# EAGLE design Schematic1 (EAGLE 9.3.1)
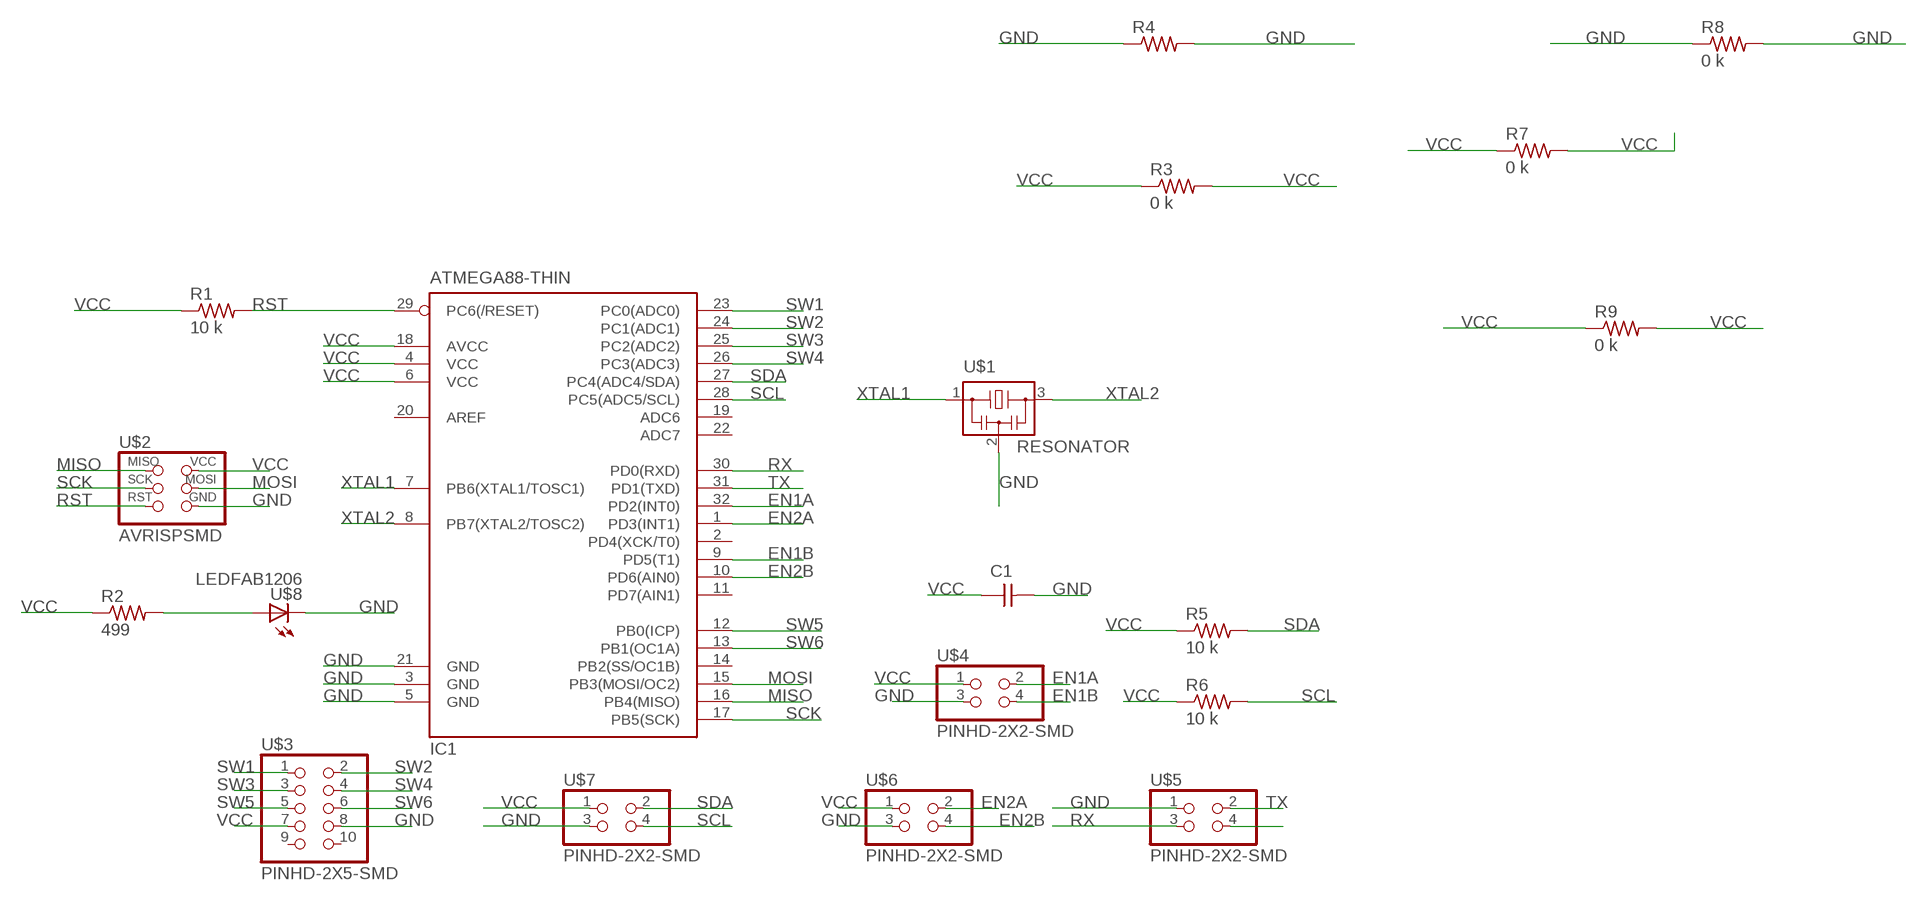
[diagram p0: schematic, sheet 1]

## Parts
C1  CAP-UNPOLARIZEDFAB  [C1206FAB]
IC1  ATMEGA88-THIN  [TQFP32-08THIN]
R1  10 k  RES-US1206FAB  [R1206FAB]
R2  499  RES-US1206FAB  [R1206FAB]
R3  0 k  RES-US1206FAB  [R1206FAB]
R4  RES-US1206FAB  [R1206FAB]
R5  10 k  RES-US1206FAB  [R1206FAB]
R6  10 k  RES-US1206FAB  [R1206FAB]
R7  0 k  RES-US1206FAB  [R1206FAB]
R8  0 k  RES-US1206FAB  [R1206FAB]
R9  0 k  RES-US1206FAB  [R1206FAB]
U$1  RESONATOR  [EFOBM]
U$2  AVRISPSMD  [2X03SMD]
U$3  PINHD-2X5-SMD  [2X05SMD]
U$4  PINHD-2X2-SMD  [2X02SMD]
U$5  PINHD-2X2-SMD  [2X02SMD]
U$6  PINHD-2X2-SMD  [2X02SMD]
U$7  PINHD-2X2-SMD  [2X02SMD]
U$8  LEDFAB1206  [LED1206FAB]

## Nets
EN1A: IC1.32(PD2(INT0)) U$4.2
EN1B: IC1.9(PD5(T1)) U$4.4
EN2A: IC1.1(PD3(INT1)) U$6.2
EN2B: IC1.10(PD6(AIN0)) U$6.4
GND: C1.2 IC1.3(GND) IC1.5(GND) IC1.21(GND) R4.1 R4.2 R8.1 R8.2 U$1.2 U$2.6(GND) U$3.8 U$4.3 U$5.1 U$6.3 U$7.3 U$8.2(C)
MISO: IC1.16(PB4(MISO)) U$2.1(MISO)
MOSI: IC1.15(PB3(MOSI/OC2)) U$2.4(MOSI)
N$1: R2.2 U$8.1(A)
N$16: U$5.4
RST: IC1.29(PC6(/RESET)) R1.2 U$2.5(RST)
RX: IC1.30(PD0(RXD)) U$5.3
SCK: IC1.17(PB5(SCK)) U$2.3(SCK)
SCL: IC1.28(PC5(ADC5/SCL)) R6.2 U$7.4
SDA: IC1.27(PC4(ADC4/SDA)) R5.2 U$7.2
SW1: IC1.23(PC0(ADC0)) U$3.1
SW2: IC1.24(PC1(ADC1)) U$3.2
SW3: IC1.25(PC2(ADC2)) U$3.3
SW4: IC1.26(PC3(ADC3)) U$3.4
SW5: IC1.12(PB0(ICP)) U$3.5
SW6: IC1.13(PB1(OC1A)) U$3.6
TX: IC1.31(PD1(TXD)) U$5.2
VCC: C1.1 IC1.4(VCC) IC1.6(VCC) IC1.18(AVCC) R1.1 R2.1 R3.1 R3.2 R5.1 R6.1 R7.1 R7.2 R9.1 R9.2 U$2.2(VCC) U$3.7 U$4.1 U$6.1 U$7.1
XTAL1: IC1.7(PB6(XTAL1/TOSC1)) U$1.1
XTAL2: IC1.8(PB7(XTAL2/TOSC2)) U$1.3
Unconnected: IC1.2(PD4(XCK/T0)) IC1.11(PD7(AIN1)) IC1.14(PB2(SS/OC1B)) IC1.19(ADC6) IC1.20(AREF) IC1.22(ADC7) U$3.9 U$3.10

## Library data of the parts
C1 = fab:CAP-UNPOLARIZED
IC1 = fab:ATMEGA88-THIN
R1-R9 = fab:RES-US: Resistor (US Symbol)
U$1 = fab:RESONATOR
U$2 = fab:AVRISP
U$3 = fab:PINHD-2X5-SMD
U$4-U$7 = fab:PINHD-2X2-SMD
U$8 = fab:LED: LED

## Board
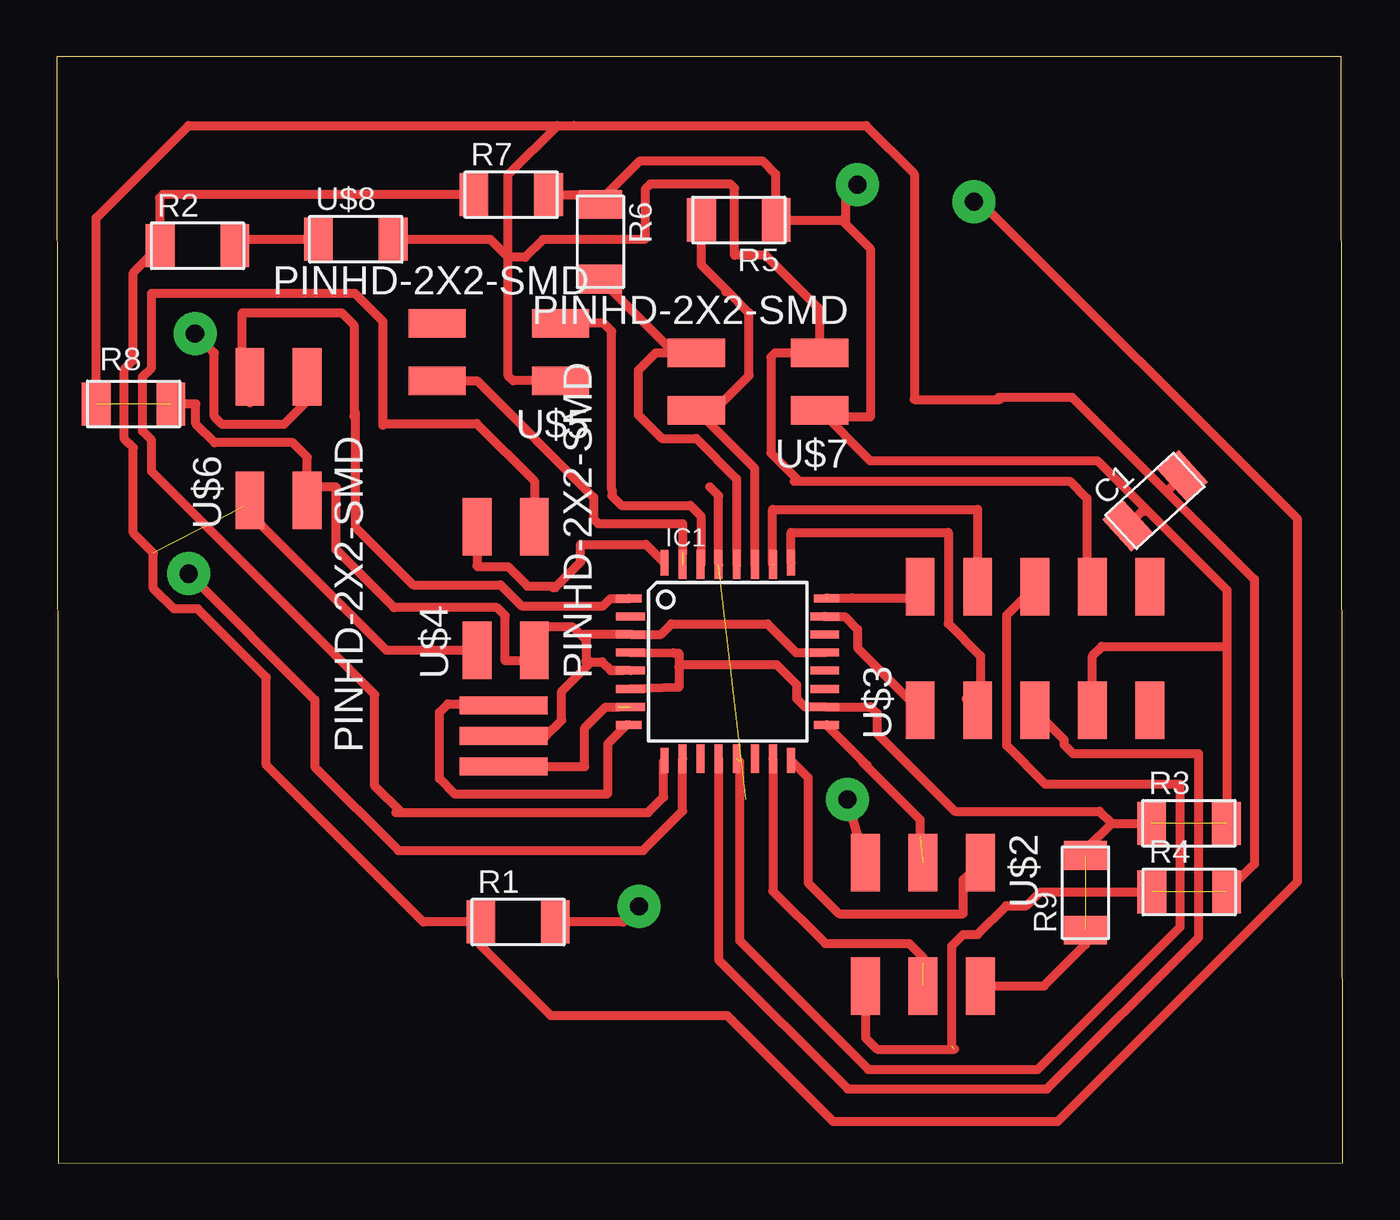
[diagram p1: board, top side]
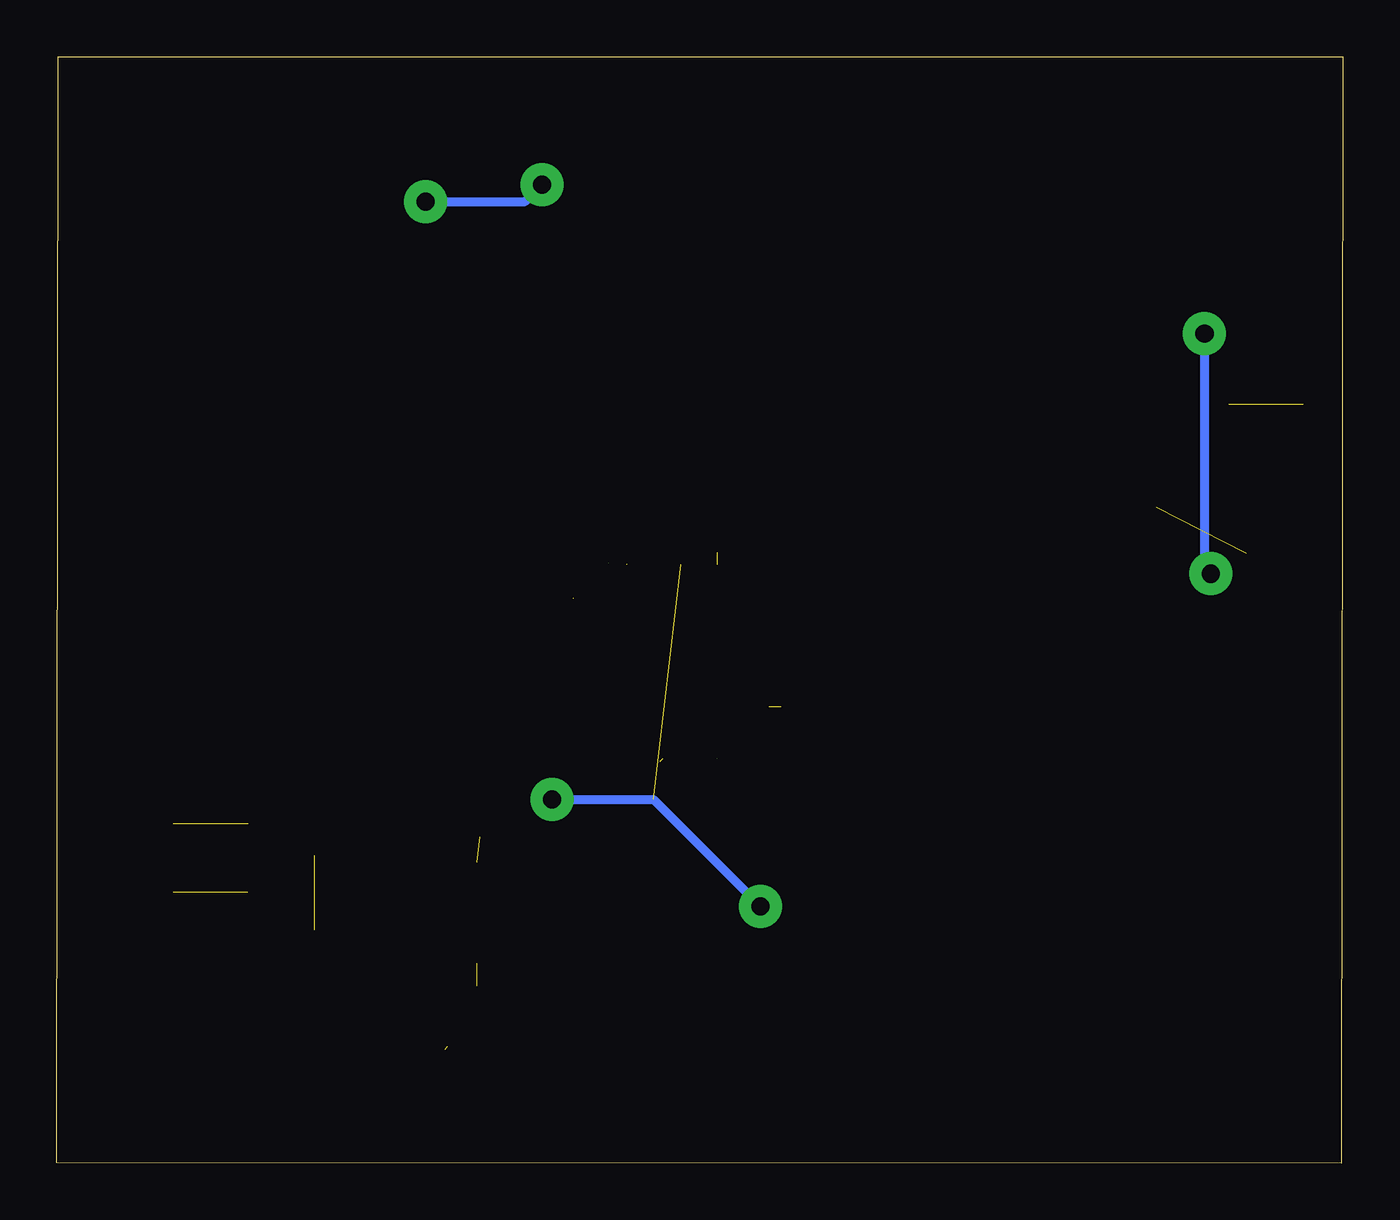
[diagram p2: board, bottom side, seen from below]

Size 56.89 x 48.95 mm. Coordinates in mm from the lower left corner, seen from the top.
Outline: 0.08,0 56.89,0.01 56.81,48.95 0,48.93 0.08,0
Copper layers (1*16): Top 0.035mm / dielectric 1.5mm / Bottom 0.035mm
Design rules "default *": minimum track width 16mil, minimum drill 0.35mm, track to track 16mil, track to pad 16mil, pad to pad 16mil, via to via 16mil, smd to smd 16mil, copper to edge 40mil, drill to drill 6mil, minimum pad ring 10mil, minimum via ring 8mil, stop-mask expansion 4mil, vias tented up to drill 0mil, thermal gap 10mil

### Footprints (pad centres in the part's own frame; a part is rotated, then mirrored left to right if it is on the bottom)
C1206FAB = smd 1.27 x 1.905: 1 -1.651,0; 2 1.651,0
TQFP32-08THIN = smd 1.118 x 0.356: 1 -4.369,2.8; 8 -4.369,-2.8; 17 4.369,-2.8; 24 4.369,2.8 | smd 1.27 x 0.356: 2 -4.293,2; 3 -4.293,1.2; 4 -4.293,0.4; 5 -4.293,-0.4; 6 -4.293,-1.2; 7 -4.293,-2; 18 4.293,-2; 19 4.293,-1.2; 20 4.293,-0.4; 21 4.293,0.4; 22 4.293,1.2; 23 4.293,2 | smd 0.356 x 1.118: 9 -2.8,-4.369; 16 2.8,-4.369; 25 2.8,4.369; 32 -2.8,4.369 | smd 0.356 x 1.27: 10 -2,-4.293; 14 1.2,-4.293; 15 2,-4.293; 26 2,4.293; 27 1.2,4.293; 31 -2,4.293 | smd 0.35 x 1.27: 11 -1.2,-4.293; 12 -0.4,-4.293; 13 0.4,-4.293; 28 0.4,4.293; 29 -0.4,4.293; 30 -1.2,4.293
R1206FAB = smd 1.27 x 1.905: 1 -1.651,0; 2 1.651,0
EFOBM = smd 0.8 x 3.9: 1 -1.35,0; 2 0,0; 3 1.35,0
2X03SMD = smd 2.54 x 1.27: 1 -2.54,2.54; 2 2.92,2.54; 3 -2.54,0; 4 2.92,0; 5 -2.54,-2.54; 6 2.92,-2.54
2X05SMD = smd 2.54 x 1.27: 1 -2.54,2.54; 2 2.92,2.54; 3 -2.54,0; 4 2.92,0; 5 -2.54,-2.54; 6 2.92,-2.54; 7 -2.54,-5.08; 8 2.92,-5.08; 9 -2.54,-7.62; 10 2.92,-7.62
2X02SMD = smd 2.54 x 1.27: 1 -2.54,1.27; 2 2.92,1.27; 3 -2.54,-1.27; 4 2.92,-1.27
LED1206FAB = smd 1.27 x 1.905: 1 -1.651,0; 2 1.651,0

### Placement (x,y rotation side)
C1  48.58,29.3 42.4 top
IC1  29.68,22.19 0 top
R1  20.41,10.67 0 top
R2  6.24,40.58 0 top
R3  50.08,15.04 0 top
R4  50.09,12 0 top
R5  30.18,41.72 180 top
R6  24.05,40.75 270 top
R7  20.1,42.84 0 top
R8  3.4,33.58 0 top
R9  45.5,11.96 90 top
U$1  19.77,18.9 90 top
U$2  38.32,10.76 270 top
U$3  40.73,22.57 90 top
U$4  19.86,25.23 90 top
U$5  19.75,35.88 180 top
U$6  9.82,31.86 90 top
U$7  31.22,34.57 180 top
U$8  13.23,40.87 0 top

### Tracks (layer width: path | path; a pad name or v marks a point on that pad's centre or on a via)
EN1A
  Top 0.406: 18.52,28.23 U$4.2 18.59,26.43 18.63,26.39 19.96,26.39 20.83,25.53 21.91,25.53 21.97,25.46 22.05,25.46 23.18,26.59 23.18,27.37 26.07,27.37 IC1.32 | IC1.32
EN1B
  Top 0.406: IC1.9 26.85,17.79 26.85,16.19 26.16,15.51 15.25,15.51 | 15,15.51 15.25,15.51 | 15.25,15.51 14.07,16.69 14.07,20.73 4.2,30.59 4.2,31.98 3.81,32.37 3.81,34.78 4.2,35.18 4.2,38.48 13.18,38.48 14.43,37.24 14.43,32.63 14.52,32.71 18.58,32.71 21.13,30.16 U$4.4
EN2A
  Top 0.406: IC1.1 25.3,24.97 24.5,24.97 24.18,24.65 20.55,24.65 19.63,25.58 15.77,25.58 13.21,28.14 13.21,32.98 | 13.21,33.18 13.21,32.98 | 8.55,33.63 U$6.2 8.22,35.11 8.22,37.62 12.6,37.62 13.16,37.06 13.16,33.03 13.21,32.98
EN2B  (via drill 0.8 pad 1.9)  (1 unrouted)
  Top 0.406: 27.69,17.89 27.69,15.58 25.95,13.83 15.13,13.83 11.42,17.54 11.42,20.5 v5.84,26.07 | U$6.4 11.09,33.72 10.05,32.68 7.33,32.68 6.97,33.03 6.97,35.84 v6.12,36.69
  Bottom 0.406: v6.12,36.69 6.12,26.35 v5.84,26.07
GND  (3 unrouted)
  Top 0.406: IC1.21 32.71,22.59 31.44,23.85 27.19,23.85 26.73,23.39 IC1.3 23.44,23.39 | U$2.6 35.78,5.55 36.28,5.04 39.71,5.04 | 39.59,5.17 39.59,9.61 40.09,10.12 40.73,10.12 42,11.39 42.89,11.39 43.5,12 R4.1 | 24.51,21.79 24.52,21.79 25.03,21.79 | IC1.5 24.51,21.79 | 23.63,22.17 23.43,22.17 23.41,22.2 23.41,23.14 | 23.63,22.17 24.12,22.17 24.51,21.79 | 23.44,23.39 23.37,23.39 | 23.44,23.39 23.41,23.35 23.41,23.14 | 32.63,30.16 32.84,30.16 | 32.84,30.16 44.81,30.16 45.57,29.4 45.57,25.73 U$3.8 | 51.74,12.6 R4.2 52.97,13.23 52.97,25.82 49.02,29.77 | U$7.3 34.11,35.84 | 49.02,29.77 44.92,33.87 41.67,33.87 41.58,33.78 | 23.41,23.14 22.83,23.71 21.6,23.71 21.13,23.24 U$4.3 20.66,22.22 19.84,22.22 19.84,24.22 19.48,24.57 14.92,24.57 12.36,27.13 12.36,29.88 12.38,29.9 11.66,29.9 U$6.3 11.09,31.23 10.45,31.86 6.99,31.86 6.16,32.7 6.16,33.58 R8.2 | 23.63,22.17 22.33,20.87 22.33,19.59 21.64,18.9 U$1.2 | U$5.1 20.19,34.61 19.98,34.82 19.98,40.07 | 19.98,40.07 19.98,43.73 22.15,45.9 | U$7.3 31.78,35.84 31.58,35.65 31.58,31.42 32.84,30.16 | 22.15,45.9 22.89,45.9 35.8,45.9 37.93,43.76 37.93,33.78 41.58,33.78 | 41.58,33.78 41.72,33.78 | C1.2 49.16,29.77 49.02,29.77 | U$7.3 33.76,37.76 31.36,40.16 30,40.16 29.98,40.17 29.98,43.12 29.79,43.31 26.26,43.31 26.03,43.08 26.03,40.88 26.01,40.86 21.51,40.86 20.73,40.07 19.98,40.07 | U$8.2 19.18,40.87 19.98,40.07 | R8.1 1.75,41.81 5.84,45.9 22.15,45.9
MISO
  Top 0.406: IC1.16 33.24,17.06 33.24,12.41 34.61,11.04 40.09,11.04 40.09,12.53 U$2.1
MOSI  (1 unrouted)
  Top 0.406: IC1.15 31.68,12.04 34,9.72 37.7,9.72 38.32,9.11 38.32,8.85
N$1
  Top 0.406: R2.2 8.18,40.87 U$8.1
RST  (via drill 0.8 pad 1.9)  (1 unrouted)
  Top 0.406: U$2.5 v34.97,16.09 | v25.76,11.35 25.07,10.67 R1.2 | IC1.29 29.28,29.52 28.89,29.91
  Bottom 0.406: v34.97,16.09 30.49,16.09 v25.76,11.35
RX
  Top 0.406: 28.5,26.49 28.5,26.5 | U$5.3 24.19,37.15 24.55,36.79 24.55,29.8 24.56,29.79 24.56,29.51 24.98,29.1 28.03,29.1 28.5,28.63 28.5,26.49 | 28.5,26.49 IC1.30
SCK  (1 unrouted)
  Top 0.406: 35.65,17.78 35.65,17.74 35.84,17.55 | 38.19,14.44 38.19,15.2 35.84,17.55 | IC1.17 35.84,17.6 35.84,17.55
SCL
  Top 0.406: IC1.28 30.08,30.27 28.3,32.05 26.77,32.05 25.72,33.11 25.72,35.06 26.49,35.84 U$7.4 27.32,35.84 R6.2
SDA
  Top 0.406: IC1.27 30.88,30.72 U$7.2 29.1,33.3 30.63,34.84 30.63,37.6 29.64,38.59 | 29.64,38.59 29.59,38.54 | 29.64,38.59 28.52,39.71 R5.2
SW1
  Top 0.406: IC1.23 33.98,24.17 34.86,24.17 35.43,23.61 35.43,22.79 U$3.1
SW2  (1 unrouted)
  Top 0.406: 34.05,25 35.18,25 | 35.18,25 35.2,24.99 | 35.18,25 37.7,25 U$3.2
SW3  (1 unrouted)
  Top 0.406: 40.22,20.54 U$3.3 40.86,20.15 40.86,22.44 39.43,23.86 39.43,27.9 32.48,27.9 IC1.25
SW4  (1 unrouted)
  Top 0.406: 41.11,26.5 40.73,26.12 | 40.73,26.12 U$3.4 | 40.73,26.12 40.73,28.92 31.67,28.92 31.67,26.48
SW5
  Top 0.406: IC1.12 29.28,9 34.99,3.29 43.8,3.29 50.51,9.99 50.51,18.11 44.96,18.11 44.56,18.5 44.56,18.73 U$3.5
SW6  (1 unrouted)
  Top 0.406: 30.21,17.77 30.21,9.85 35.9,4.15 43.39,4.15 49.69,10.45 49.69,16.76 43.74,16.76 42.02,18.48 42.02,24.24 U$3.6 43.14,25.36
TX  (1 unrouted)
  Top 0.406: 27.69,27 27.69,28.28 23.96,28.28 23.75,28.5 23.75,29.45 18.59,34.61 U$5.2
VCC  (via drill 0.8 pad 1.9)  (3 unrouted)
  Top 0.406: IC1.4 27.27,22.57 27.52,22.57 27.52,21.93 | IC1.6 27.52,21.04 27.52,21.93 | 27.52,21.93 27.65,22.06 31.84,22.06 32.73,21.17 32.73,20.56 33.08,20.2 33.19,20.2 | 33.19,20.2 33.23,20.16 | 33.19,20.2 33.96,20.2 IC1.18 36,20.19 36.28,19.9 36.28,19.01 39.73,15.57 46.13,15.57 46.66,15.04 | 46.19,19.65 U$3.7 45.81,22.45 46.21,22.86 51.75,22.86 | 46.66,15.04 R3.1 | 48.26,28.84 46.02,31.08 35.98,31.08 U$7.1 34.05,33.01 35.99,33.01 35.99,40.45 34.89,41.55 | 48.26,28.84 51.75,25.35 51.75,22.86 | 51.75,22.86 51.75,15.04 R3.2 | 34.89,41.55 34.72,41.72 R5.1 31.8,41.74 31.8,43.75 31.22,44.34 25.81,44.34 24.05,42.58 24.05,42.43 | C1.1 48.01,28.84 48.26,28.84 | R6.1 24.05,42.43 | R7.2 23.65,42.84 24.05,42.43 | R7.1 4.71,42.84 4.56,42.68 4.56,39.73 4.43,39.73 4.58,39.88 R2.1 3.39,39.38 3.39,35.51 3,35.12 3,32.04 3.39,31.64 3.39,27.88 4.28,26.98 4.28,25.43 5.2,24.51 6.25,24.51 9.27,21.49 9.27,17.61 16.22,10.67 R1.1 18.76,9.64 21.86,6.54 29.65,6.54 34.34,1.85 44.27,1.85 54.89,12.47 54.89,28.49 40.84,42.53 v40.56,42.53 | U$4.1 14.58,22.69 8.25,29.03 U$6.1 | U$2.2 43.66,7.84 45.5,9.68 R9.1 | v35.42,43.28 34.89,42.75 34.89,41.55 | 46.66,15.04 45.5,13.88 R9.2
  Bottom 0.406: v40.56,42.53 36.17,42.53 v35.42,43.28
XTAL1  (1 unrouted)
  Top 0.406: 24.85,20.17 24.28,20.17 23.36,19.25 23.36,17.55 U$1.1
XTAL2
  Top 0.406: 25.23,19.4 25.3,19.4 IC1.8 25.22,19.39 24.37,18.54 24.37,16.36 24.33,16.32 17.63,16.32 16.93,17.02 16.93,19.94 17.31,20.32 19.7,20.32 U$1.3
